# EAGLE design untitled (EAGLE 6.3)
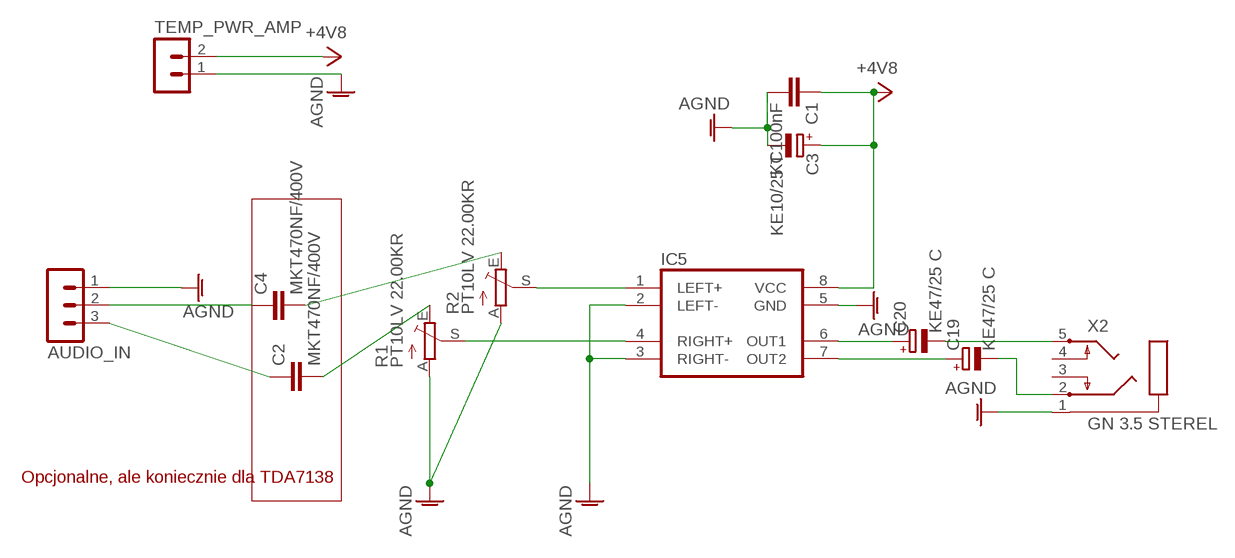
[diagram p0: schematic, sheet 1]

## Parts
AUDIO_IN  MA03-1  [MA03-1]
C1  KC100nF  C-EU025-025X050  [C025-025X050]
C2  MKT470NF/400V  C-EU150-091X182  [C150-091X182]
C3  KE10/25 T  CPOL-EUTT2D6  [TT2D6]
C4  MKT470NF/400V  C-EU150-091X182  [C150-091X182]
C19  KE47/25 C  CPOL-EUD  [PANASONIC_D]
C20  KE47/25 C  CPOL-EUD  [PANASONIC_D]
IC5  TDA7050  [DIL08]
R1  PT10LV 22.00KR  TRIM_EU-CA9V  [CA9V]
R2  PT10LV 22.00KR  TRIM_EU-CA9V  [CA9V]
TEMP_PWR_AMP  MA02-1  [MA02-1]
X2  GN 3.5 STEREL  STEREOJACK  [STX3100]

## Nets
+5V: C1.1 C3.+ IC5.8(VCC) TEMP_PWR_AMP.2 ; supply symbol labelled +4V8
AGND: AUDIO_IN.1 C1.2 C3.- IC5.2(LEFT-) IC5.3(RIGHT-) IC5.5(GND) R1.A R2.A TEMP_PWR_AMP.1 X2.1
N$1: AUDIO_IN.3 C2.1
N$2: AUDIO_IN.2 C4.1
N$7: IC5.1(LEFT+) R2.S
N$10: C2.2 R1.E
N$11: C4.2 R2.E
N$20: IC5.4(RIGHT+) R1.S
N$21: C19.+ IC5.7(OUT2)
N$22: C20.+ IC5.6(OUT1)
N$23: C19.- X2.2
N$24: C20.- X2.5
Unconnected: X2.3 X2.4

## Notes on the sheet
- Opcjonalne, ale koniecznie dla TDA7138

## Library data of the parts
AUDIO_IN = con-lstb:MA03-1: PIN HEADER; OC_FARNELL: unknown; OC_NEWARK: unknown
C1 C2 C4 = rcl:C-EU: CAPACITOR, European symbol
C3 C19 C20 = rcl:CPOL-EU: POLARIZED CAPACITOR, European symbol
IC5 = tda7050:TDA7050
R1 R2 = pot:TRIM_EU-: POTENTIOMETER
TEMP_PWR_AMP = con-lstb_SileliS:MA02-1: PIN HEADER
X2 = adafruit:STEREOJACK: MIC/HEADPHONE JACK Stereo jack with two switches. Kycon STX3100, CUI SJ1-3555NG and/or 4UCon 05544

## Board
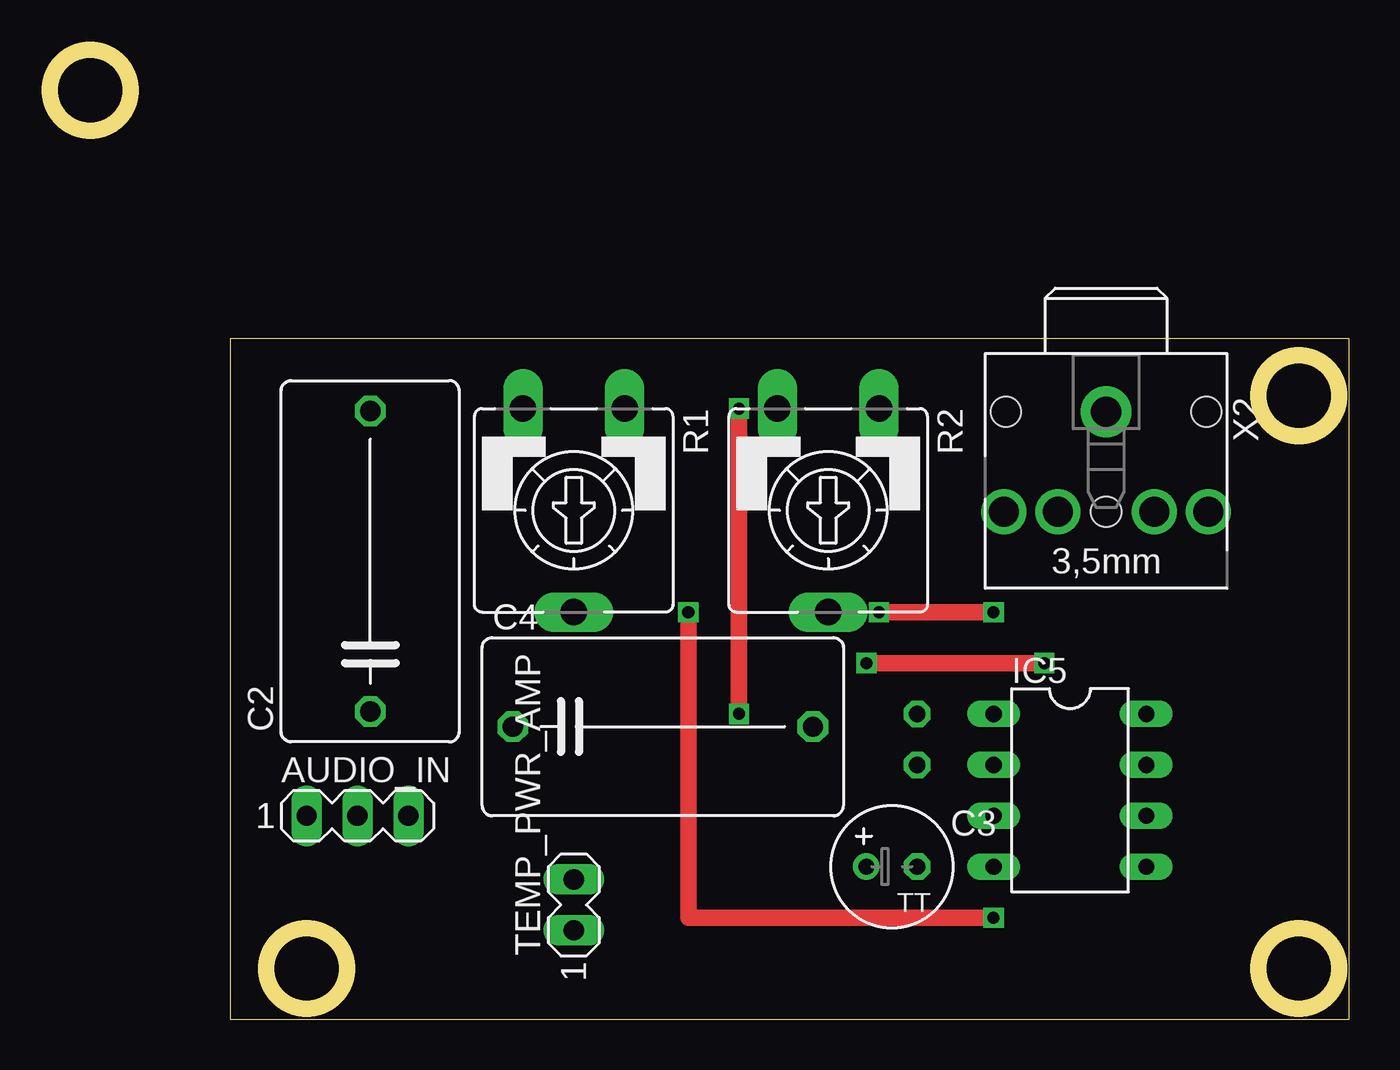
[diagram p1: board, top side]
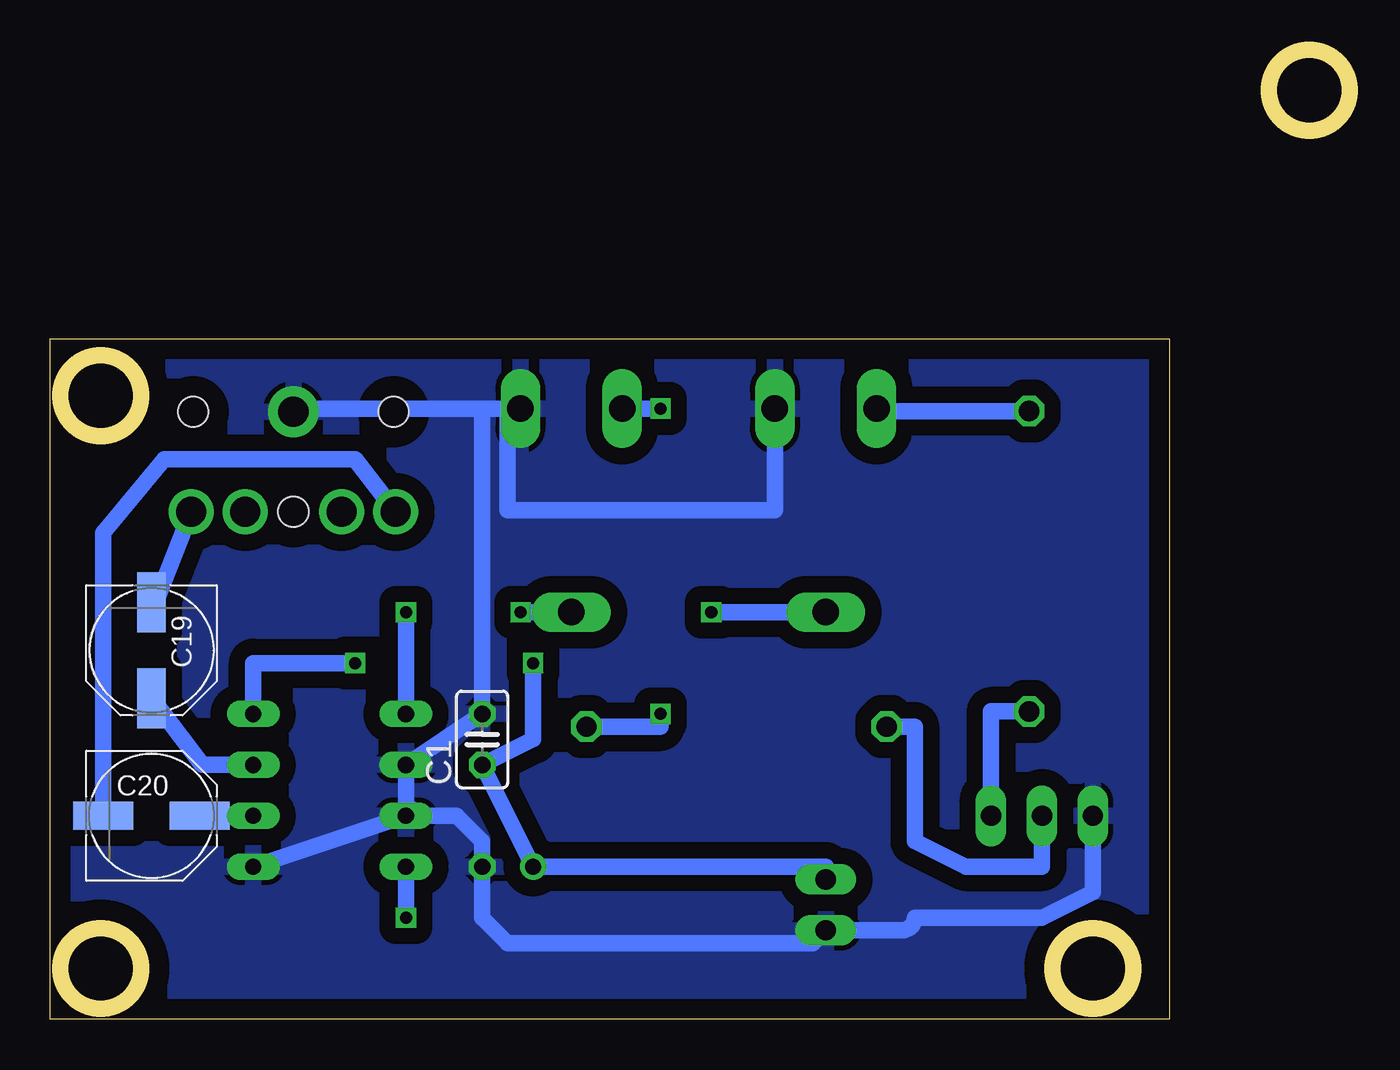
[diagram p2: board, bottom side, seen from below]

Size 64.85 x 48.36 mm. Coordinates in mm from the lower left corner, seen from the top.
Outline: 8.99,0 64.85,0 64.85,33.96 8.99,33.96 8.99,0
Outline: circle at 2.01,46.36 radius 2.01
Outline: circle at 62.33,31.11 radius 2.01
Outline: circle at 62.33,2.54 radius 2.01
Outline: circle at 12.8,2.54 radius 2.01
Copper layers (1*16): Top 0.035mm / dielectric 1.5mm / Bottom 0.035mm
Design rules "default": minimum track width 10mil, minimum drill 24mil, track to track 8mil, track to pad 8mil, pad to pad 8mil, via to via 8mil, smd to smd 8mil, copper to edge 40mil, drill to drill 8mil, minimum pad ring 10mil, minimum via ring 8mil, stop-mask expansion 4mil, vias tented up to drill 0mil, thermal gap 10mil

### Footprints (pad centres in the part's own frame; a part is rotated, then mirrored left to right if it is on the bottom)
MA03-1 = drill 1.016 long: 1 -2.54,0; 2 0,0; 3 2.54,0
C025-025X050 = drill 0.813 octagon: 1 -1.27,0; 2 1.27,0
C150-091X182 = drill 1.016 octagon: 1 -7.493,0; 2 7.493,0
TT2D6 = drill 0.813: + -1.27,0 | drill 0.813 octagon: - 1.27,0
PANASONIC_D = smd 3 x 1.4: + 2.4,0; - -2.4,0
DIL08 = drill 0.813 long: 1 -3.81,-3.81; 2 -1.27,-3.81; 3 1.27,-3.81; 4 3.81,-3.81; 5 3.81,3.81; 6 1.27,3.81; 7 -1.27,3.81; 8 -3.81,3.81
CA9V = drill 1.321 long: A -2.54,-5.08; E 2.54,-5.08; S 0,5.08
MA02-1 = drill 1.016 long: 1 -2.54,0; 2 0,0
STX3100 = drill 1.5 pad 2.54: 1 2.7,-0.1 | drill 1.5: 2 7.7,5; 3 7.7,2.3; 4 7.7,-2.5; 5 7.7,-5.2 | hole 1.5: 2.7,4.9; 2.7,-5.1; 7.7,-0.1

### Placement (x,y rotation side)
AUDIO_IN  15.34,10.16 0 top
C1  43.28,13.97 90 bottom
C2  15.98,22.86 90 top
C3  42.01,7.62 0 top
C4  30.58,14.61 0 top
C19  59.79,18.41 270 bottom
C20  59.79,10.16 0 bottom
IC5  50.9,11.43 270 top
R1  26.14,25.4 180 top
R2  38.84,25.4 180 top
TEMP_PWR_AMP  26.14,6.98 90 top
X2  52.81,33.02 270 top

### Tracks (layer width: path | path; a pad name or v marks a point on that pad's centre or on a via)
+5V  (via drill 0.6)
  Top 0.813: v49.63,17.78 v40.74,17.78
  Bottom 0.813: IC5.8 54.71,17.78 v49.63,17.78 | v40.74,17.78 40.74,13.97 C1.1 C3.+ 26.14,7.62 TEMP_PWR_AMP.2
AGND
  Bottom 0.813: IC5.3 46.77,10.48 | R2.A 42.01,30.48 | 42.01,30.48 43.28,30.48 | 43.28,30.48 52.55,30.48 arc-90 X2.1 | 43.28,30.48 C1.2 IC5.2 IC5.3 | AUDIO_IN.1 12.8,6.35 15.34,5.08 21.69,5.08 arc90 22.33,4.45 TEMP_PWR_AMP.1 26.77,3.81 42.01,3.81 43.28,5.08 C3.- 43.28,8.89 44.55,10.16 IC5.3 | IC5.3 IC5.5 | R1.A 28.68,25.4 42.01,25.4 42.01,30.48
  pour Bottom (isolate 0.813): 6.45,36.83 67.41,36.83 67.41,-2.54 6.45,-2.54
N$1
  Bottom 0.813: C2.1 17.88,15.37 AUDIO_IN.3
N$2
  Bottom 0.813: C4.1 21.69,14.61 21.69,8.89 19.15,7.62 15.34,7.62 AUDIO_IN.2
N$7  (via drill 0.6)
  Top 0.813: v47.09,20.32 v41.38,20.32
  Bottom 0.813: IC5.1 v47.09,20.32 | v41.38,20.32 R2.S
N$10
  Bottom 0.813: C2.2 23.6,30.35 R1.E
N$11  (via drill 0.6)
  Top 0.813: v34.39,15.24 v34.39,30.48
  Bottom 0.813: C4.2 34.39,14.61 v34.39,15.24 | v34.39,30.48 R2.E
N$20  (via drill 0.6)
  Top 0.813: v47.09,5.08 31.85,5.08 v31.85,20.32
  Bottom 0.813: IC5.4 v47.09,5.08 | v31.85,20.32 R1.S
N$21
  Bottom 0.813: IC5.7 57.25,12.7 C19.+
N$22
  Bottom 0.813: IC5.6 C20.+
N$23
  Bottom 0.813: X2.2 59.79,20.32 C19.-
N$24
  Bottom 0.813: X2.5 49.63,27.94 59.16,27.94 62.19,24.27 C20.-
